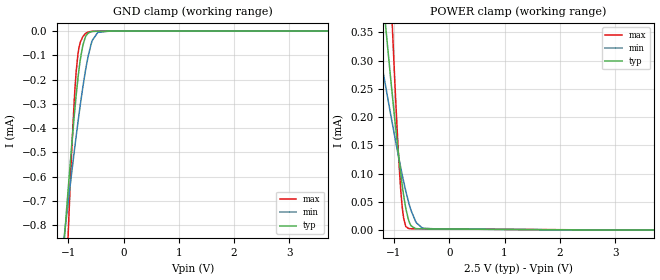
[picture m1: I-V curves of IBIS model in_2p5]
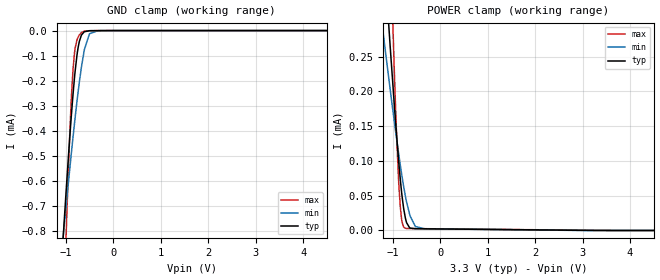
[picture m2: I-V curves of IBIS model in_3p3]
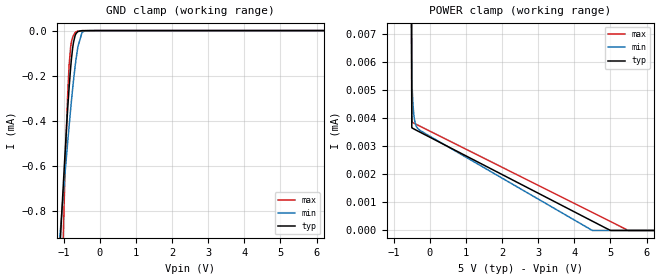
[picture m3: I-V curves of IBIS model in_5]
|Texas Instruments Incorporated
| High-Performance, 8000 VPK Reinforced Dual Channel Digital Isolator
| Marketing part#   Digital Voltage Range   Package-type   #pins
| ISO7820FDW   2.25V-5.5V   SOIC   16
| ISO7820FDWW   2.25V-5.5V   SOIC   16
[IBIS Ver]   4.1
[File name]   iso7820f.ibs
[File Rev]   1.1
[Date]   5/12/2016
[Source]
| Texas Instruments Incorporated.
| Analog-eLab Design Center, HPA
| 12500 TI Blvd
| Dallas, TX -75243
[Notes]   Revision History:
| Rev 1.1: 5/12/2016
| - Add DWW package component
| Rev 1.0: 7/2/2015
| - Initial version of the model
| - Model generated from simulations in TISPICE
| - Model matched to SPICE simulation
| - C_comp although listed in numerical order of value are
|   obtained from varying PVT conditions. For PVT conditions for
|   each specific value refer the buffer description under
|   respective [Model]. IBIS model user is responsible for using
|   appropriate C_comp to simulate for Signal Integrity.
| - This is relative part of ISO7841F.
|* EXCEPTION:   *
|* - For in_* models there will be leakage current in POWER clamp   *
|*   because of a resistor(R1) connected to pad.   *
[Disclaimer]
| This model is designed as an aid for customers of Texas Instruments.
| TI and its licensors and suppliers make no warranties, either expressed
| or implied, with respect to this  model, including the warranties of
| merchantability or fitness for a particular purpose. The model is
| provided solely on an "as is" basis. The entire risk as to its quality
| and performance is with the customer.
[Copyright]
(C) Copyright 2016 Texas Instruments Incorporated.All rights reserved.
|   IS07820FDW
[Component]   IS07820FDW
[Manufacturer]   TI
[Package]   |16 SOIC - DW package
|   typ   min   max
R_pkg   0.12558   0.1249   0.12620
L_pkg   1.93563nH   1.9245nH   1.94750nH
C_pkg   0.4209pF   0.3263pF   0.6128pF
[Pin]  signal_name   model_name   R_pin   L_pin   C_pin
1   GND1   GND   0.0970   2.2582nH   0.6389pF
2   NC   NC   0.1057   2.1519nH   0.3071pF
3   VCC1   POWER   0.1289   1.9955nH   0.2145pF
4   INA   IN   0.1250   1.9245nH   0.3778pF
5   INB   IN   0.1249   1.9265nH   0.3667pF
6   NC   NC   0.1404   2.1876nH   0.4324pF
7   GND1   GND   0.1781   2.8364nH   0.4590pF
8   NC   NC   0.0822   2.4395nH   0.4450pF
9   GND2   GND   0.1013   2.4407nH   0.4093pF
10   NC   NC   0.1793   2.8571nH   0.5272pF
11   NC   NC   0.1288   1.9962nH   0.5084pF
12   OUTB   OUT   0.1262   1.9440nH   0.3263pF
13   OUTA   OUT   0.1262   1.9475nH   0.6128pF
14   VCC2   POWER   0.1405   2.1861nH   0.3810pF
15   NC   NC   0.0827   2.0901nH   0.7509pF
16   GND2   GND   0.0975   2.2691nH   0.6744pF
|   IS07820FDWW
[Component]   IS07820FDWW
[Manufacturer]   TI
[Package]   |16 SOIC - DWW package
|   typ   min   max
R_pkg   0.2986   0.2007   0.3729
L_pkg   6.1920nH   5.7068nH   6.9814nH
C_pkg   0.3776pF   0.0527pF   0.7658pF
[Pin]  signal_name   model_name   R_pin   L_pin   C_pin
1   GND1   GND   0.2515   6.9814nH   0.7658pF
2   NC   NC   0.2414   6.4743nH   0.4827pF
3   VCC1   POWER   0.3404   6.2419nH   0.3712pF
4   INA   IN   0.2997   5.8575nH   0.3661pF
5   INB   IN   0.3048   5.7068nH   0.3697pF
6   NC   NC   0.3229   5.9972nH   0.3885pF
7   GND1   GND   0.3729   6.6301nH   0.3885pF
8   NC   NC   0.2162   5.8346nH   0.4827pF
9   GND2   GND   0.2007   6.5823nH   0.5517pF
10   NC   NC   0.3456   6.8632nH   0.3887pF
11   NC   NC   0.3109   6.1891nH   0.3704pF
12   OUTB   OUT   0.2997   5.7473nH   0.3669pF
13   OUTA   OUT   0.3032   5.8251nH   0.3710pF
14   VCC2   POWER   0.3351   6.1684nH   0.0527pF
15   NC   NC   0.2007   5.7509nH   0.5517pF
16   GND2   GND   0.2768   6.8945nH   0.0527pF
|   Model Selectors
[Model Selector] IN
in_2p5   2.5V digital Input
in_3p3   3.3V digital Input
in_5   5.0V digital Input
[Model Selector] OUT
out_2p5   2.5V digital 3-state
out_3p3   3.3V digital 3-state
out_5   5.0V digital 3-state
| Models and submodels in the file (6): in_2p5 (Input), in_3p3 (Input), in_5 (Input), out_2p5 (3-state), out_3p3 (3-state), out_5 (3-state)
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|   in_2p5 Model
[Model]   in_2p5
Model_type   Input
Vinl = 0.75
Vinh = 1.75
|   typ   min   max
|   (nom PVT)   (fast PVT)   (slow PVT)
C_comp   3.281e-15   3.281e-15   3.250e-14
[Model spec]
|subparameter
Vinl   0.75   0.675   0.825
Vinh   1.75   1.575   1.925
| Where nom  PVT is Nominal Process, 2.5V, 27C
|   Fast PVT is Strong Process,  2.75V, -55C
|   Slow PVT is Weak Process,   2.25V, 150C
[Voltage Range]   2.5   2.25   2.75
|Junction Temperature
[Temperature Range]   27   150   -55
[Power Clamp Reference]   2.5   2.25   2.75
[GND Clamp Reference]   0   0   0
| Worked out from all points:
|   GND clamp passes 1 mA (typ) near -1.12 V on its own axis
[GND Clamp]
|   Voltage   I(typ)   I(min)   I(max)
-2.5V     -5.567mA   -3.855mA   -11.2mA
-1.069V   -852.9uA   -838.7uA   -1.235mA
-1.015V   -691.7uA   -732.3uA   -913.4uA
-962.5mV  -540.3uA   -630.7uA   -621.5uA
-880mV    -320.6uA   -475.8uA   -242.7uA
-825mV    -195.8uA   -377.3uA   -96.08uA
-735mV    -57.68uA   -229.6uA   -22.57uA
-641mV    -8.597uA   -105.1uA   -3.988uA
-564mV    -1.717uA   -38.11uA   -871.4nA
-466mV    -415.4nA   -5.597uA   -322nA
-250mV    -166.5nA   -222.7nA   -161.2nA
5V        0A         0A         0A
[POWER Clamp]
|   Voltage   I(typ)   I(min)   I(max)
-2.5V     1.814mA    1.041mA    3.986mA
-1.351V   566.8uA    365.9uA    1.114mA
-1.196V   405.7uA    279uA      742.4uA
-1.053V   260.5uA    200.3uA    408.8uA
-990.2mV  199.2uA    166.7uA    271uA
-924.3mV  138.4uA    132.7uA    141.2uA
-874.8mV  96.55uA    108.3uA    65.49uA
-822.5mV  58.5uA     83.91uA    18.88uA
-740mV    18.48uA    50.19uA    2.683uA
-612.5mV  2.435uA    15.71uA    2.168uA
-486.3mV  1.99uA     3.311uA    2.086uA
5V        0A         0A         0A
|   in_3p3 Model
[Model]   in_3p3
Model_type   Input
Vinl = 0.99
Vinh = 2.31
|   typ   min   max
|   (nom PVT)   (fast PVT)   (slow PVT)
C_comp   3.281e-15   3.281e-15   3.329e-14
[Model spec]
|subparameter
Vinl   0.99   0.891   1.089
Vinh   2.31   2.079   2.541
| Where nom  PVT is Nominal Process, 3.3V, 27C
|   Fast PVT is Strong Process,  3.63V, -55C
|   Slow PVT is Weak Process,   2.97V, 150C
[Voltage Range]   3.3   2.97   3.63
|Junction Temperature
[Temperature Range]   27   150   -55
[Power Clamp Reference]   3.3   2.97   3.63
[GND Clamp Reference]   0   0   0
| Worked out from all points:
|   GND clamp passes 1 mA (typ) near -1.12 V on its own axis
|   POWER clamp passes 1 mA (typ) near -1.75 V on its own axis
[GND Clamp]
|   Voltage   I(typ)   I(min)   I(max)
-3.3V     -8.284mA   -5.57mA    -16.97mA
-1.076V   -873.6uA   -852.3uA   -1.277mA
-1.002V   -654.2uA   -707.4uA   -840.1uA
-891.3mV  -349uA     -496.6uA   -285.5uA
-853.4mV  -257.3uA   -427.5uA   -158.6uA
-821.7mV  -189.1uA   -371.5uA   -90.58uA
-768.9mV  -98.39uA   -282.7uA   -37.63uA
-719.4mV  -43.62uA   -206.4uA   -17.63uA
-617.1mV  -5.129uA   -80.39uA   -2.416uA
-505.2mV  -641.2nA   -12.81uA   -412.3nA
-330mV    -221.3nA   -470.3nA   -212.8nA
6.6V      0A         0A         0A
[POWER Clamp]
|   Voltage   I(typ)   I(min)   I(max)
-3.3V     2.696mA    1.52mA     6.012mA
-1.242V   453.3uA    304.9uA    851.4uA
-1.198V   407.7uA    280.3uA    746.3uA
-1.049V   257.2uA    198.7uA    400.8uA
-965.9mV  176.8uA    154.6uA    221.3uA
-878.8mV  100.3uA    110.8uA    71.18uA
-842.5mV  72.63uA    93.56uA    33uA
-805.2mV  48.41uA    76.82uA    11.74uA
-737.2mV  18.14uA    49.73uA    3.193uA
-526mV    2.561uA    5.724uA    2.679uA
-330mV    2.416uA    2.488uA    2.553uA
6.6V      0A         0A         0A
|   in_5 Model
[Model]   in_5
Model_type   Input
Vinl = 1.5
Vinh = 3.5
|   typ   min   max
|   (nom PVT)   (fast PVT)   (slow PVT)
C_comp   3.281e-15   3.281e-15   3.455e-14
[Model spec]
|subparameter
Vinl   1.5   1.35   1.65
Vinh   3.5   3.15   3.85
| Where nom  PVT is Nominal Process, 5V, 27C
|   Fast PVT is Strong Process,  5.5V, -55C
|   Slow PVT is Weak Process,   4.5V, 150C
[Voltage Range]   5   4.5   5.5
|Junction Temperature
[Temperature Range]   27   150   -55
[Power Clamp Reference]   5   4.5   5.5
[GND Clamp Reference]   0   0   0
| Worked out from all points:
|   GND clamp passes 1 mA (typ) near -1.12 V on its own axis
[GND Clamp]
|   Voltage   I(typ)   I(min)   I(max)
-5V       -13.99mA   -9.044mA   -29.25mA
-1.112V   -984.3uA   -924.5uA   -1.502mA
-1.062V   -831.8uA   -824.9uA   -1.192mA
-974mV    -572.9uA   -652.8uA   -683.2uA
-908mV    -391.9uA   -527.5uA   -354.9uA
-850mV    -249.6uA   -421.5uA   -149.8uA
-809mV    -164.5uA   -349.6uA   -72.24uA
-740mV    -62.8uA    -237.2uA   -24.38uA
-608mV    -4.229uA   -71.85uA   -2.005uA
-500mV    -598.4nA   -11.5uA    -395.2nA
-347mV    -233.9nA   -591nA     -223.9nA
10V       0A         0A         0A
[POWER Clamp]
|   Voltage   I(typ)   I(min)   I(max)
-5V       185.5mA    66.86mA    305.6mA
-1.007V   217uA      177.2uA    308.5uA
-500mV    3.667uA    5.488uA    3.869uA
-486.5mV  3.656uA    5.003uA    3.86uA
-468.5mV  3.642uA    4.538uA    3.848uA
-428mV    3.613uA    3.98uA     3.822uA
-374mV    3.577uA    3.716uA    3.787uA
-279.5mV  3.514uA    3.578uA    3.726uA
4.5V      333.1nA    0A         645nA
5.005V    0A         0A         319.1nA
5.49V     0A         0A         0A
10V       0A         0A         0A
